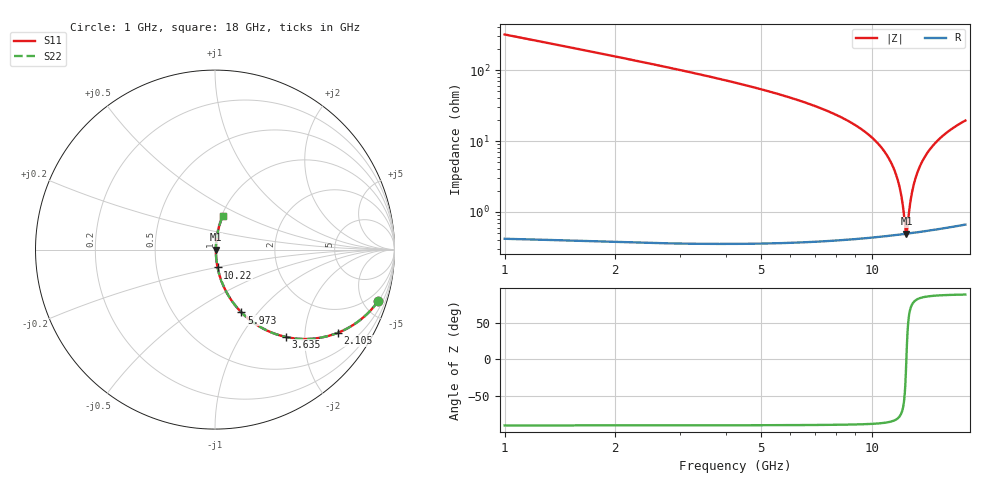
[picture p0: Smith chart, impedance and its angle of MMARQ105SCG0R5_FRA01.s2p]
! MMARQ105SCG0R5_FRA01  S-PARAMETER MODEL  ( General Type )
! Model Generated by TAIYO YUDEN Corporation (http://www.ty-top.com)
! Version 1.0
! TAIYO YUDEN Control No. 200326
! Copyright(c) 2020 TAIYO YUDEN CO.,LTD. All Rights Reserved.
! Product Description (link to TY-COMPAS)
! https://ds.yuden.co.jp/TYCOMPAS/or/detail?pn=MMARQ105SCG0R5BFRA01&u=M
! Products Name : Multilayer Ceramic Capacitors
! Characteristics :
!  Capacitance : 0.5 pF , Rated Voltage : 250V , TCC : CG / C0G
!  Case Size : 1.0 x 0.5 / 0.039 x 0.02 [mm/inch] , Thickness : 0.5 / 0.02 [mm/inch]
!  (Conditions: Temperature = 25 degC , DC Bias Current/Voltage = 0A / 0V)
! External Node Assignments :
!  1  o---| |---o  2
! GND o---------o GND
! Frequency Range : 1GHz  -  18GHz  [ 401 STEP ]
# MHz S RI R 50
! Freq[MHz].  S11 Real  S11 Imag  S21 Real  S21 Imag  S12 Real  S12 Imag  S22 Real  S22 Imag
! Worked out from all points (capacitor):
!   401 points, 1 GHz to 18 GHz, reference 50 ohm
!   read as one part in series: C = 497 fF near 1.085 GHz
!   lowest |Z| = 494 mohm at 12.43 GHz (marker M1)
!   series resonance near 12.43 GHz, so ESL is about 330 pH
!   S11 on the Smith chart (normalised r, x): 1 GHz: 1.01, -6.36; 2.105 GHz: 1.01, -2.95; 3.635 GHz: 1.01, -1.61; 5.973 GHz: 1.01, -0.82; 10.22 GHz: 1.01, -0.20; 18 GHz: 1.01, +0.39
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1000  0.9096 -0.286  0.0904 0.286  0.0904 0.286  0.9096 -0.286
1552.5  0.8041 -0.3959  0.1959 0.3959  0.1959 0.3959  0.8041 -0.3959
2105  0.6851 -0.4632  0.3149 0.4632  0.3149 0.4632  0.6851 -0.4632
3635  0.3937 -0.4864  0.6063 0.4864  0.6063 0.4864  0.3937 -0.4864
3847.5  0.3619 -0.4782  0.6381 0.4782  0.6381 0.4782  0.3619 -0.4782
5972.5  0.1474 -0.35  0.8526 0.35  0.8526 0.35  0.1474 -0.35
6695  0.1059 -0.3022  0.8941 0.3022  0.8941 0.3022  0.1059 -0.3022
9500  0.0232 -0.1362  0.9768 0.1362  0.9768 0.1362  0.0232 -0.1362
10222.5  0.0144 -0.0993  0.9856 0.0993  0.9856 0.0993  0.0144 -0.0993
11072.5  0.00806 -0.0589  0.9919 0.0589  0.9919 0.0589  0.00806 -0.0589
11667.5  0.00576 -0.0322  0.9942 0.0322  0.9942 0.0322  0.00576 -0.0322
12050  0.00506 -0.0158  0.9949 0.0158  0.9949 0.0158  0.00506 -0.0158
12347.5  0.0049 -0.00339  0.9951 0.00339  0.9951 0.00339  0.0049 -0.00339
12432.5  0.00491 0.000107  0.9951 -0.000107  0.9951 -0.000107  0.00491 0.000107
12517.5  0.00494 0.00358  0.9951 -0.00358  0.9951 -0.00358  0.00494 0.00358
12687.5  0.00509 0.0104  0.9949 -0.0104  0.9949 -0.0104  0.00509 0.0104
12857.5  0.00532 0.0172  0.9947 -0.0172  0.9947 -0.0172  0.00532 0.0172
13070  0.00574 0.0256  0.9943 -0.0256  0.9943 -0.0256  0.00574 0.0256
13325  0.00641 0.0354  0.9936 -0.0354  0.9936 -0.0354  0.00641 0.0354
14090  0.00946 0.0637  0.9905 -0.0637  0.9905 -0.0637  0.00946 0.0637
15195  0.0162 0.1016  0.9838 -0.1016  0.9838 -0.1016  0.0162 0.1016
18000  0.0423 0.185  0.9577 -0.185  0.9577 -0.185  0.0423 0.185
